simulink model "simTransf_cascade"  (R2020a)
settings: Solver=ode15s  StartTime=0.0  StopTime=tsim  FixedStep=0.1  MaxStep=1  RelTol=1e-5
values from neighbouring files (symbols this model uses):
  C = Fc*cpc/(Fh*cph)    [calcblock.m]    (also in calcblock2.m; calcblock3.m; calcv0.m; eNTU.m = m.c*cp.c/(m.h*cp.h))
  d_tstep = [500; 50000; 70000; 130000; 50000; 50000]    [runTransf.m]    (also in runTransfOL.m = [500 5000 7000 13000]; Main.m = [1000; 1000;2000]; Main_OL.m = 300; runTestCalcBlk.m = 300)
  dFh = 2    [runTransf.m]    (also in runTransfOL.m = 0; Main.m = 0;0.2*Fh)
  dTcin = 0    [runTransf.m]    (also in runTransfOL.m; Main.m = 2)
  dThin = 0    [runTransf.m]    (also in runTransfOL.m; Main.m = 0;2)
  dU = U0*0    (= 0)    [runTransf.m]    (also in runTransfOL.m)
  dvsp = dvsp_vec(i)    [runTransf.m]    (also in runTransfOL.m = [0;0];vsp0*0)
  Fc0 = 5    [runTransf.m]    (also in runTransfOL.m; Main.m; Main_OL.m; runTestCalcBlk.m)
  Fh = d(1)    [calcblock.m]    (also in calcblock2.m; calcblock3.m; calcblockv2.m; calcv0.m)
  Kc = 1/kM(i)*tau(i)/(tauCM(i)+theta(i))    [runTransf.m]    (also in runTransfOL.m; Main.m = 1/k*tau/(tauC+theta))
  KI = 1/kS(i)*1/tauCS(i)    [runTransf.m]    (also in runTransfOL.m; Main.m = Kp/tauIv; Main_OL.m = 1)
  nd = size(d0,1)    [runTransf.m]    (also in runTransfOL.m = size(d0,2); Main.m = size(d0,2); Main_OL.m = size(d0,2); runTestCalcBlk.m = size(d0,2))
  np = size(p,2)    [runTransf.m]    (also in runTransfOL.m; runH2Psim.m = length(param); Main.m; Main_OL.m)
  nu = 1    [runTransf.m]    (also in runTransfOL.m; runH2Psim.m = length(u0); Main.m; Main_OL.m)
  nx = size(x0,1)    [runTransf.m]    (also in runTransfOL.m; H2P_Turbine_driven.m = param(end); runTD.m = length(x0); H2P_Boiler_driven.m = param(end))
  p = [U;A;Fc(i);Fh;cpc;cph;Tcin;Thin]    [NonlinearMap.m]    (also in runTransf.m = [N, Fc0, rhoc, rhoh, U0, A,cpc,cph]; runTransfOL.m = [N, Fc0, rhoc, rhoh, U0, A,cpc,cph]; Main.m = [N, Fc0, rhoc, rhoh,U,A,cpc,cph]; Main_OL.m = [N, Fc0, rhoc, rhoh,U,A,cpc,cph])
  tauI = min(tau(i), 4*(tauCM(i)+theta(i)))    [runTransf.m]    (also in runTransfOL.m; Main.m = min(tau,4*(tauC+theta)))
  Tcin = d(2)    [calcblock.m]    (also in calcblock2.m; calcblock3.m; calcblockv2.m; calcv0.m)
  Thin = d(3)    [calcblock.m]    (also in calcblock2.m; calcblock3.m; calcblockv2.m; calcv0.m)
  Thsp = Thsp0    [runTransf.m]    (also in runTransfOL.m; Main.m = Thsp0+dThsp; Main_OL.m = Thsp0+dThsp; runTestCalcBlk.m = Thsp0+dThsp)
  Thsp0 = x0(end-1);  2.971202611676064e+02    [runTransf.m]    (also in runTransfOL.m = x0(end);  2.971202611676064e+02; Main.m = Thend(end); Main_OL.m = 297.120261168; runTestCalcBlk.m = Thend(end))
  trf = i    [runTransf.m]    (also in runTransfOL.m = zeros(3,1))
  tstep = 10000    [runTransf.m]    (also in runTransfOL.m = 100; Main_OL.m = 100; Main.m = 100)
  U0 = 150    [runTransf.m]    (also in runTransfOL.m)
  vsp0 = vsp0_vec(i)    [runTransf.m]    (also in runTransfOL.m = [v00; Thin + (Fc0* cpc)/(Fh*cph)*(Tcin-x0(1)); Fc0*(Tcin-x0()
  x0 = [Tcend(1:N)'; Thend(1:N)';Thin]    [runTransf.m]    (also in runTransfOL.m = [Tcend(1:N)'; Thend(1:N)']; runTD.m = [TE0;TD0;TSh0;MD0; MSh0;w0;TA0;0;0;0;0;0;0;0;0;0]; runBD.m = [TE0;TD0;TSh0;MD0; MSh0;w0;TA0;0;0;0;0;0;0;0;0;0]; runFP.m = [TE0;TD0;TSh0;MD0; MSh0;w0;TA0;0;0;0;0;0;0;0])
undefined symbols (not defined in the file or in its folder): calcv0, calcv2, calcvE, HEXode, i

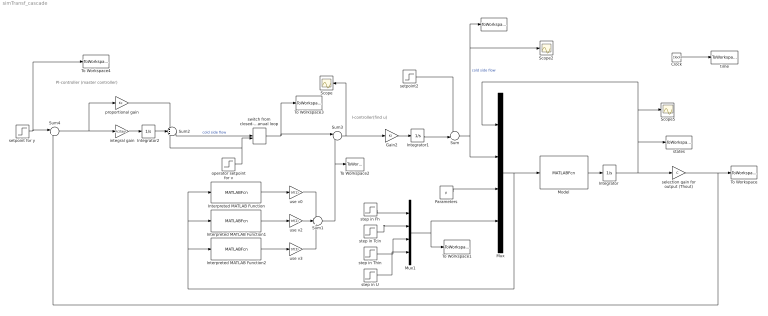
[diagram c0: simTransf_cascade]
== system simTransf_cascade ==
  note: I-controller(find u)
  note: PI-controller (master controller)
  " " : ToWorkspace  VariableName=u  SampleTime=-1
  Clock : Clock
  Gain2 : Gain  Gain=KI  Multiplication=Matrix(K*u)
  "Integrator " : Integrator  InitialCondition=x0
  Integrator1 : Integrator
  Integrator2 : Integrator
  Interpreted MATLAB Function : MATLABFcn  MATLABFcn=calcv0(u(1:nx),u(nx+1:nx+nu),u(nx+nu+1:nx+nu+np),u(nx+nu+np+1:nx+nu+np+nd))  OutputDimensions=1
  Interpreted MATLAB Function1 : MATLABFcn  MATLABFcn=calcv2(u(1:nx),u(nx+1:nx+nu),u(nx+nu+1:nx+nu+np),u(nx+nu+np+1:nx+nu+np+nd))  OutputDimensions=1
  Interpreted MATLAB Function2 : MATLABFcn  MATLABFcn=calcvE(u(1:nx),u(nx+1:nx+nu),u(nx+nu+1:nx+nu+np),u(nx+nu+np+1:nx+nu+np+nd))  OutputDimensions=1
  Model : MATLABFcn  MATLABFcn=HEXode(u(1:nx),u(nx+1:nx+nu),u(nx+nu+1:nx+nu+np),u(nx+nu+np+1:nx+nu+np+nd))  OutputDimensions=nx  Output1D=off
  Mux : Mux
  Mux1 : Mux
  Parameters : Constant  Value=p
  Scope : Scope
  Scope2 : Scope
  Scope5 : Scope
  Sum : Sum  Inputs=++|
  Sum1 : Sum  Inputs=+++
  Sum2 : Sum  Inputs=+++
  Sum3 : Sum  Inputs=|+-
  Sum4 : Sum  Inputs=|+-
  To Workspace : ToWorkspace  VariableName=Thout  SampleTime=-1
  To Workspace1 : ToWorkspace  VariableName=d  SampleTime=-1
  To Workspace2 : ToWorkspace  VariableName=v  SampleTime=-1
  To Workspace3 : ToWorkspace  VariableName=vs  SampleTime=-1
  To Workspace4 : ToWorkspace  VariableName=ys  SampleTime=-1
  integral gain : Gain  Gain=Kc/tauI  Multiplication=Matrix(K*u)
  operator setpoint for v : Step  Time=tstep  Before=vsp0(i)  After=vsp0(i)+dvsp(i)  SampleTime=0
  proportional gain : Gain  Gain=Kc  Multiplication=Matrix(K*u)
  selection gain for output (Thout) : Gain  Gain=C  Multiplication=Matrix(K*u)
  setpoint for y : Step  Time=tstep  Before=Thsp0  After=Thsp  SampleTime=0
  setpoint2 : Step  Time=10  Before=Fc0  After=Fc0*1  SampleTime=0
  states : ToWorkspace  VariableName=y  SampleTime=-1
  step in Fh : Step  Time=d_tstep(1)  Before=Fh  After=Fh+dFh  SampleTime=0
  step in Tcin : Step  Time=d_tstep(2)  Before=Tcin  After=Tcin+dTcin  SampleTime=0
  step in Thin : Step  Time=d_tstep(3)  Before=Thin  After=Thin+dThin  SampleTime=0
  step in U : Step  Time=d_tstep(4)  Before=U0  After=U0-dU  SampleTime=0
  switch from closed-loop to manual loop : ManualSwitch  CurrentSetting=0
  time : ToWorkspace  VariableName=t  SampleTime=-1
  use v0 : Gain  Gain=trf(1)  Multiplication=Matrix(K*u)
  use v2 : Gain  Gain=trf(2)  Multiplication=Matrix(K*u)
  use v3 : Gain  Gain=trf(3)  Multiplication=Matrix(K*u)
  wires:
  Model/1 -> "Integrator "/1
  "Integrator "/1 -> selection gain for output (Thout)/1, states/1, Mux/1, Scope5/1
  Clock/1 -> time/1
  Parameters/1 -> Mux/3
  Sum/1 -> Mux/2, Scope2/1, " "/1  "cold side flow"
  selection gain for output (Thout)/1 -> Sum4/2, To Workspace/1
  switch from closed-loop to manual loop/1 -> To Workspace3/1, Sum3/1
  Mux1/1 -> Mux/4, To Workspace1/1
  step in Fh/1 -> Mux1/1
  step in Tcin/1 -> Mux1/2
  step in Thin/1 -> Mux1/3
  Gain2/1 -> Integrator1/1
  Sum3/1 -> Gain2/1, Scope/1
  setpoint2/1 -> Sum/1
  Integrator1/1 -> Sum/2
  Mux/1 -> Interpreted MATLAB Function/1, Interpreted MATLAB Function1/1, Interpreted MATLAB Function2/1, Model/1
  Interpreted MATLAB Function/1 -> use v0/1
  Sum1/1 -> To Workspace2/1, Sum3/2
  Interpreted MATLAB Function1/1 -> use v2/1
  Interpreted MATLAB Function2/1 -> use v3/1
  use v0/1 -> Sum1/1
  use v2/1 -> Sum1/2
  use v3/1 -> Sum1/3
  operator setpoint for v/1 -> switch from closed-loop to manual loop/2, Sum2/3
  Integrator2/1 -> Sum2/2
  integral gain/1 -> Integrator2/1
  proportional gain/1 -> Sum2/1
  Sum2/1 -> switch from closed-loop to manual loop/1  "cold side flow"
  Sum4/1 -> proportional gain/1, integral gain/1
  setpoint for y/1 -> To Workspace4/1, Sum4/1
  step in U/1 -> Mux1/4
